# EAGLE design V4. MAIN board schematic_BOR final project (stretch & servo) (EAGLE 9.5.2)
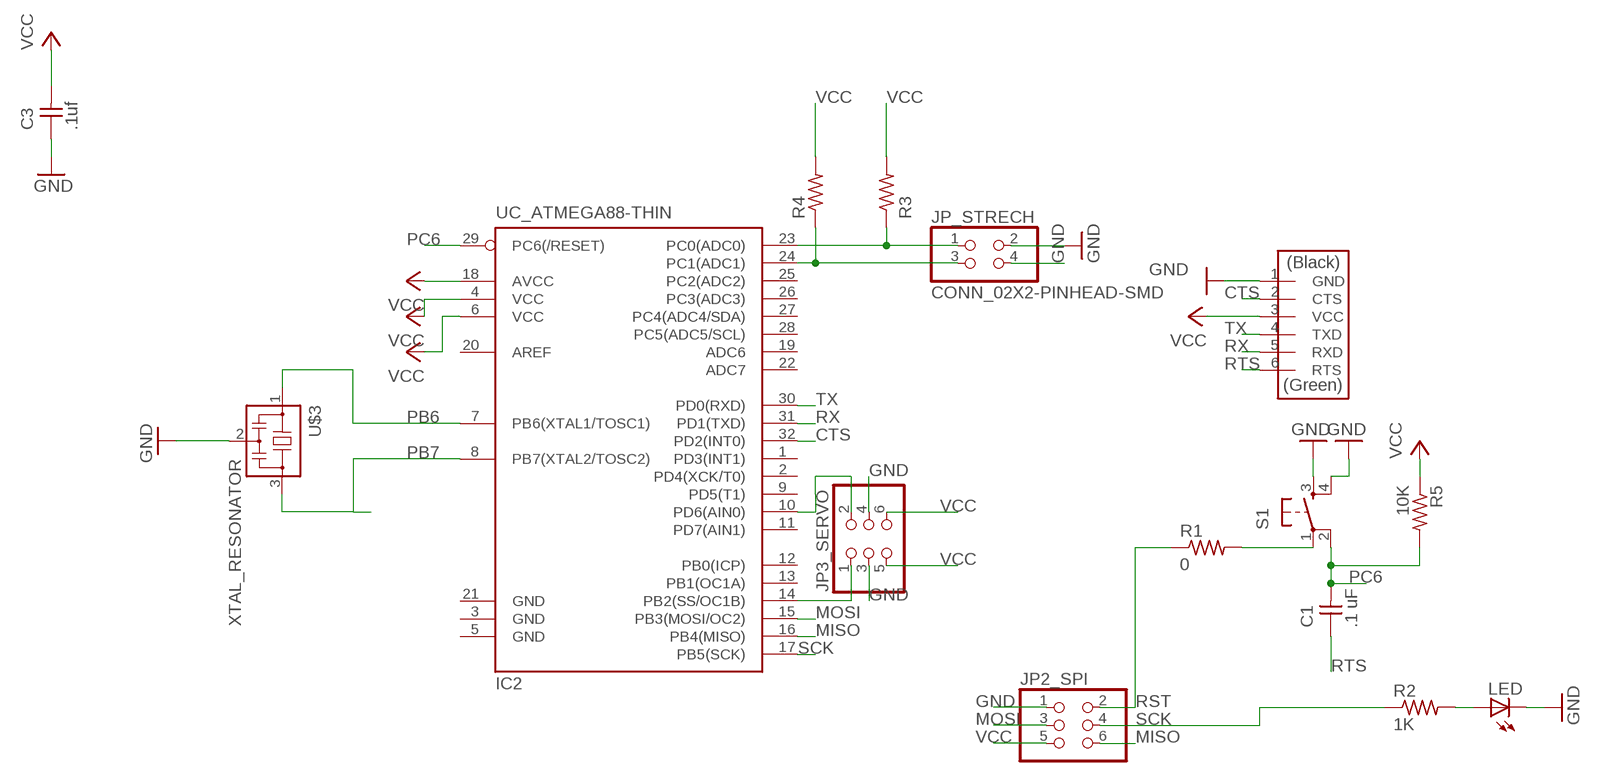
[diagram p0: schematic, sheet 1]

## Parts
C1  .1 uF  CAP_UNPOLARIZEDFAB  [C1206FAB]
C3  .1uf  UNPOLARIZED_CAPACITOR1206  [1206]
IC2  UC_ATMEGA88-THIN  [TQFP32-08THIN]
JP2_SPI  CONN_03X2-PINHEAD-SMD  [2X03SMD]
JP3_SERVO  CONN_03X2-PINHEAD-SMD  [2X03SMD]
JP_STRECH  CONN_02X2-PINHEAD-SMD  [2X02SMD]
LED  LED1206  [1206]
R1  0  R1206FAB  [R1206FAB]
R2  1K  RESISTOR1206  [1206]
R3  R1206FAB  [R1206FAB]
R4  R1206FAB  [R1206FAB]
R5  10K  RESISTOR1206  [1206]
S1  SW_SWITCH_TACTILE_6MM6MM_SWITCH  [6MM_SWITCH]
U$1  CONN_06_FTDI-SMD-HEADER  [1X06SMD]
U$3  XTAL_RESONATOR  [EFOBM]

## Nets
CTS: IC2.32(PD2(INT0)) U$1.2(CTS)
GND: C3.1 JP2_SPI.1 JP3_SERVO.3 JP3_SERVO.4 JP_STRECH.2 JP_STRECH.4 LED.2(C) S1.3(S) S1.4(S1) U$1.1(GND) U$3.2
MISO: IC2.16(PB4(MISO)) JP2_SPI.6
MOSI: IC2.15(PB3(MOSI/OC2)) JP2_SPI.3
N$1: R1.2 S1.1(P)
N$2: IC2.10(PD6(AIN0)) JP3_SERVO.2
N$3: IC2.23(PC0(ADC0)) JP_STRECH.1 R3.1
N$4: IC2.24(PC1(ADC1)) JP_STRECH.3 R4.1
N$18: IC2.14(PB2(SS/OC1B)) JP3_SERVO.1
N$23: LED.1(A) R2.2
PB6: IC2.7(PB6(XTAL1/TOSC1)) U$3.1
PB7: IC2.8(PB7(XTAL2/TOSC2)) U$3.3
PC6: C1.2 IC2.29(PC6(/RESET)) R5.2 S1.2(P1)
RST: JP2_SPI.2 R1.1
RTS: C1.1 U$1.6(RTS)
RX: IC2.31(PD1(TXD)) U$1.5(RXD)
SCK: IC2.17(PB5(SCK)) JP2_SPI.4 R2.1
TX: IC2.30(PD0(RXD)) U$1.4(TXD)
VCC: C3.2 IC2.4(VCC) IC2.6(VCC) IC2.18(AVCC) JP2_SPI.5 JP3_SERVO.5 JP3_SERVO.6 R3.2 R4.2 R5.1 U$1.3(VCC)
Unconnected: IC2.1(PD3(INT1)) IC2.2(PD4(XCK/T0)) IC2.9(PD5(T1)) IC2.11(PD7(AIN1)) IC2.12(PB0(ICP)) IC2.13(PB1(OC1A)) IC2.19(ADC6) IC2.20(AREF) IC2.22(ADC7) IC2.25(PC2(ADC2)) IC2.26(PC3(ADC3)) IC2.27(PC4(ADC4/SDA)) IC2.28(PC5(ADC5/SCL))

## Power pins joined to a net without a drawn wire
GND: IC2.3(GND) IC2.5(GND) IC2.21(GND)

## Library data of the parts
C1 = eagle_fab:CAP_UNPOLARIZED
C3 = ng:UNPOLARIZED_CAPACITOR: unpolarized_capacitor
IC2 = eagle_fab:UC_ATMEGA88-THIN
JP2_SPI JP3_SERVO = eagle_fab:CONN_03X2-PINHEAD-SMD: PIN HEADER
JP_STRECH = eagle_fab:CONN_02X2-PINHEAD-SMD
LED = ng:LED
R1 R3 R4 = eagle_fab:R: Resistor (US Symbol)
R2 R5 = ng:RESISTOR
S1 = eagle_fab:SW_SWITCH_TACTILE_6MM: OMRON SWITCH
U$1 = eagle_fab:CONN_06_FTDI-SMD-HEADER
U$3 = eagle_fab:XTAL_RESONATOR

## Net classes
0 default: clearance 0.356 mm

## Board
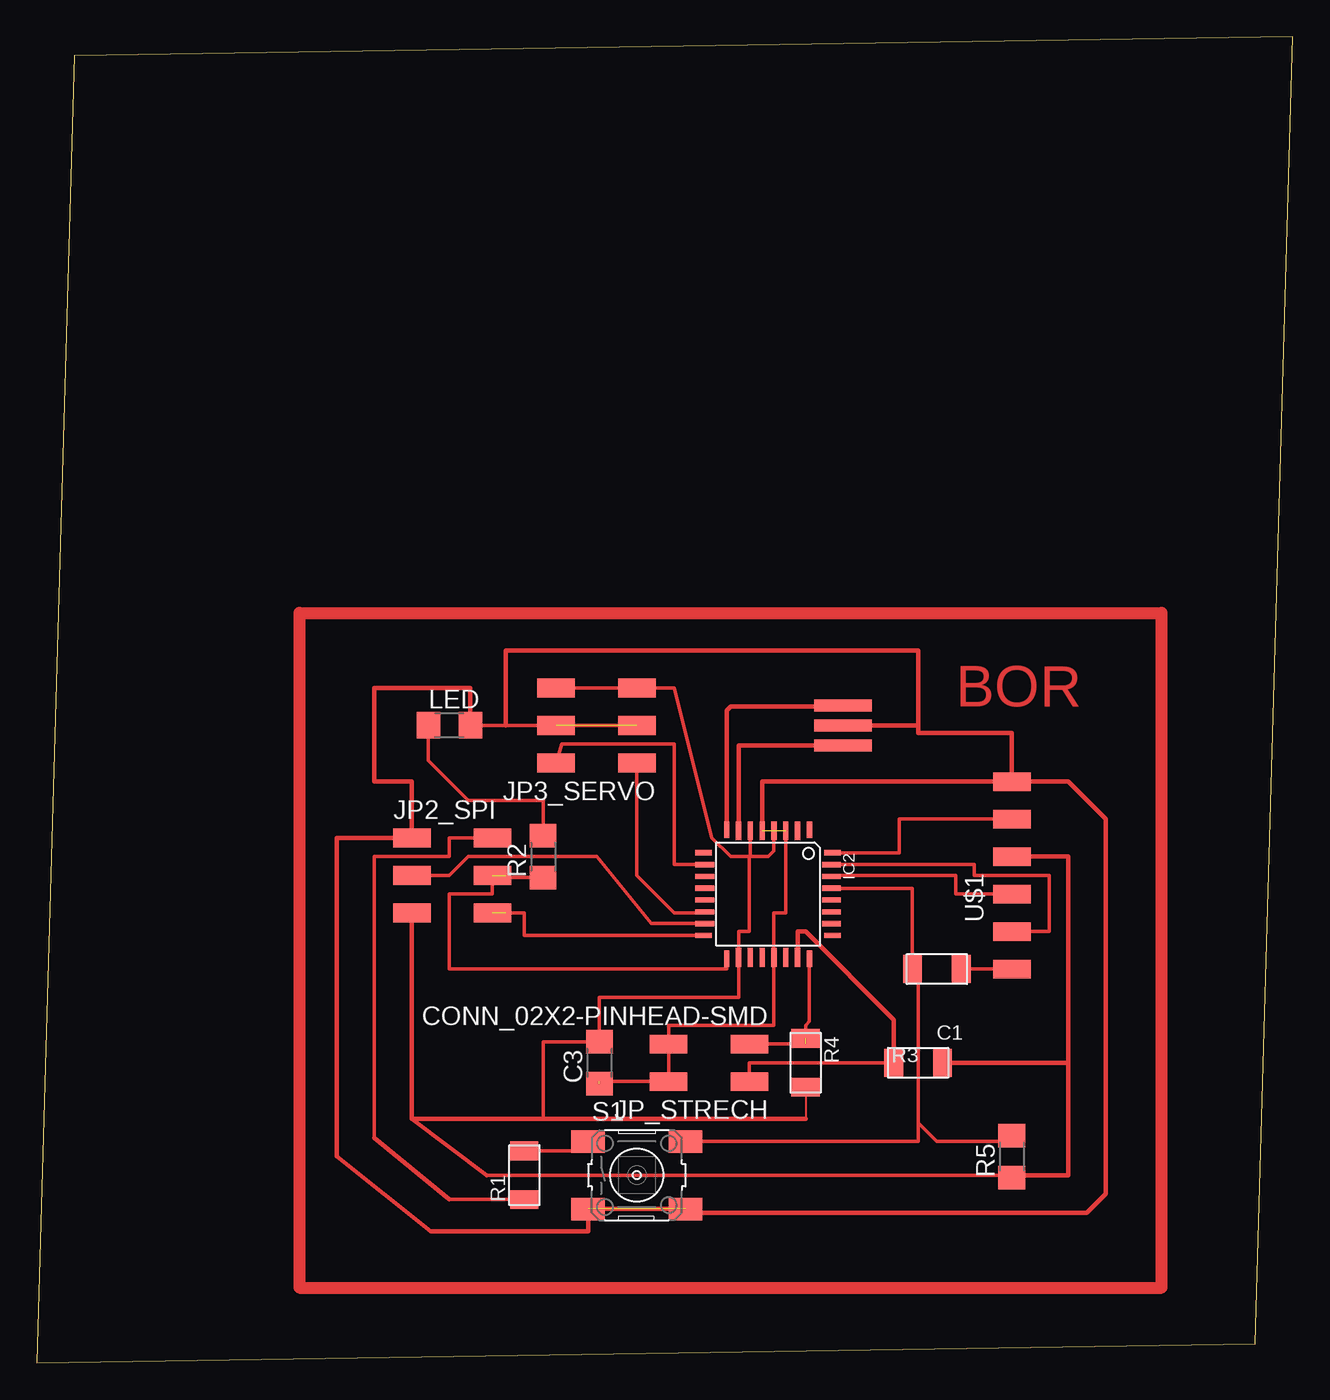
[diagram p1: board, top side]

Size 85.07 x 89.84 mm. Coordinates in mm from the lower left corner, seen from the top.
Outline: 0,0 82.53,1.27 85.07,89.84 2.54,88.57 0,0
Copper layers (1*16): Top 0.035mm / dielectric 1.5mm / Bottom 0.035mm
Design rules "default": minimum track width 6mil, minimum drill 0.35mm, track to track 6mil, track to pad 6mil, pad to pad 6mil, via to via 6mil, smd to smd 6mil, copper to edge 40mil, drill to drill 6mil, minimum pad ring 10mil, minimum via ring 8mil, stop-mask expansion 4mil, vias tented up to drill 0mil, thermal gap 10mil

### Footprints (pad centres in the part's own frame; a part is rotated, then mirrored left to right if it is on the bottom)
C1206FAB = smd 1.27 x 1.905: 1 -1.651,0; 2 1.651,0
1206 = smd 1.6 x 1.803: 1 -1.422,0; 2 1.422,0
TQFP32-08THIN = smd 1.118 x 0.356: 1 -4.369,2.8; 8 -4.369,-2.8; 17 4.369,-2.8; 24 4.369,2.8 | smd 1.27 x 0.356: 2 -4.293,2; 3 -4.293,1.2; 4 -4.293,0.4; 5 -4.293,-0.4; 6 -4.293,-1.2; 7 -4.293,-2; 18 4.293,-2; 19 4.293,-1.2; 20 4.293,-0.4; 21 4.293,0.4; 22 4.293,1.2; 23 4.293,2 | smd 0.356 x 1.118: 9 -2.8,-4.369; 16 2.8,-4.369; 25 2.8,4.369; 32 -2.8,4.369 | smd 0.356 x 1.27: 10 -2,-4.293; 14 1.2,-4.293; 15 2,-4.293; 26 2,4.293; 27 1.2,4.293; 31 -2,4.293 | smd 0.35 x 1.27: 11 -1.2,-4.293; 12 -0.4,-4.293; 13 0.4,-4.293; 28 0.4,4.293; 29 -0.4,4.293; 30 -1.2,4.293
2X03SMD = smd 2.54 x 1.27: 1 -2.54,2.54; 2 2.92,2.54; 3 -2.54,0; 4 2.92,0; 5 -2.54,-2.54; 6 2.92,-2.54
2X02SMD = smd 2.54 x 1.27: 1 -2.54,1.27; 2 2.92,1.27; 3 -2.54,-1.27; 4 2.92,-1.27
R1206FAB = smd 1.27 x 1.905: 1 -1.651,0; 2 1.651,0
6MM_SWITCH = smd 2.286 x 1.524: 1 -3.302,2.286; 2 3.302,2.286; 3 -3.302,-2.286; 4 3.302,-2.286
1X06SMD = smd 2.54 x 1.27: 1 0,6.35; 2 0,3.81; 3 0,1.27; 4 0,-1.27; 5 0,-3.81; 6 0,-6.35
EFOBM = smd 0.8 x 3.9: 1 -1.35,0; 2 0,0; 3 1.35,0

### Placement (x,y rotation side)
C1  60.96,26.67 180 top
C3  38.1,20.32 90 top
IC2  49.53,31.75 270 top
JP2_SPI  27.94,33.02 0 top
JP3_SERVO  38.1,43.18 180 top
JP_STRECH  45.72,20.32 180 top
LED  27.94,43.18 0 top
R1  33.02,12.7 90 top
R2  34.29,34.29 90 top
R3  59.69,20.32 0 top
R4  52.07,20.32 270 top
R5  66.04,13.97 90 top
S1  40.64,12.7 0 top
U$1  66.04,33.02 0 top
U$3  54.61,43.18 90 top

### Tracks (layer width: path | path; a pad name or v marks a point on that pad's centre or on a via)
CTS
  Top 0.254: U$1.2 58.42,36.83 58.42,34.55 IC2.32
GND  (4 unrouted)
  Top 0.152: 44.2,10.41 44.45,10.16
  Top 0.254: LED.2 31.75,43.18 JP3_SERVO.3 | 38.1,19.05 JP_STRECH.2 JP_STRECH.4 42.8,22.86 49.93,22.86 IC2.21 49.93,30.48 50.73,30.48 IC2.3
  Top 0.305: U$3.2 59.69,43.18 | IC2.5 49.13,39.37 U$1.1 66.04,42.67 59.69,42.67 59.69,43.18 | LED.2 29.36,45.72 22.86,45.72 22.86,39.37 25.4,39.37 JP2_SPI.1 20.32,35.56 20.32,13.97 26.67,8.89 37.34,8.89 S1.3 44.2,10.41 | 59.69,43.18 59.69,48.26 31.75,48.26 31.75,43.18 | 44.45,10.16 71.12,10.16 72.39,11.43 72.39,36.83 69.85,39.37 67.31,39.37
MISO  (1 unrouted)
  Top 0.254: IC2.16 33.02,28.95 33.02,30.48 31.75,30.48
MOSI
  Top 0.254: IC2.15 41.63,29.75 38.1,34.1 37.91,34.29 29.21,34.29 27.94,33.02 JP2_SPI.3
N$1
  Top 0.254: R1.2 37.34,14.35 S1.1
N$2
  Top 0.152: 41.91,41.91 41.91,41.89
  Top 0.254: JP3_SERVO.2 35.56,41.91 41.91,41.91 43.18,41.91 43.18,33.75 IC2.10
N$3  (1 unrouted)
  Top 0.152: 58.19,20.55 R3.1 | 58.15,20.49 57.98,20.32
  Top 0.254: JP_STRECH.1 48.26,20.32 57.98,20.32 | IC2.23 51.53,27.21
  Top 0.305: R3.1 58.04,23.24 52.07,29.21 51.53,29.21 IC2.23
N$4  (1 unrouted)
  Top 0.254: 52.07,21.59 JP_STRECH.3 | IC2.24 52.33,23.12 52.07,22.86 R4.1
N$5
  Top 0.813: 17.78,50.8 76.2,50.8 76.2,5.08 17.78,5.08 17.78,50.8
N$18
  Top 0.152: IC2.14 45.17,30.48
  Top 0.254: 45.17,30.48 43.18,30.48 40.64,33.02 JP3_SERVO.1
N$23
  Top 0.254: R2.2 34.29,38.1 29.21,38.1 26.52,40.79 LED.1
PB6
  Top 0.305: U$3.1 47.53,41.83 IC2.7
PB7
  Top 0.152: U$3.3 54.53,44.45
  Top 0.305: 54.53,44.45 46.99,44.45 46.73,44.19 IC2.8
PC6
  Top 0.152: 59.69,16.26 59.66,16.23 | 66.04,14.99 R5.2
  Top 0.254: 59.69,16.26 59.69,14.99 S1.2 | 59.69,16.26 60.96,14.99 66.04,14.99 | IC2.29 59.31,32.15 C1.2 59.69,26.67 59.69,16.26
RST
  Top 0.254: JP2_SPI.2 27.94,35.56 27.94,34.29 22.86,34.29 22.86,15.24 | 27.94,11.05 R1.1
  Top 0.305: 22.86,15.24 27.94,11.05
RTS
  Top 0.254: C1.1 U$1.6
RX
  Top 0.254: IC2.31 63.5,33.75 63.5,33.02 68.58,33.02 68.58,29.21 U$1.5
SCK  (1 unrouted)
  Top 0.152: 31.75,32.87 31.75,33.02
  Top 0.254: JP2_SPI.4 30.86,31.75 27.94,31.75 27.94,26.67 46.73,26.67 IC2.17 | R2.1 31.75,32.87
TX
  Top 0.152: IC2.30 53.82,33.02
  Top 0.254: 53.82,33.02 62.23,33.02 62.23,31.75 U$1.4
VCC
  Top 0.152: R4.2 52.07,16.51 | 66.19,12.7 R5.1 65.89,12.7
  Top 0.254: IC2.4 49.93,34.69 49.53,34.29 48.33,34.29 | 48.26,34.29 48.26,29.21 47.53,29.21 IC2.18 47.53,24.74 38.1,24.74 C3.2 34.29,21.74 34.29,16.51 | JP3_SERVO.6 JP3_SERVO.5 43.18,45.72 45.72,35.56 46.99,34.29 48.26,34.29 | 30.48,12.7 65.89,12.7 | IC2.6 48.33,34.29 | 48.33,34.29 48.26,34.29
  Top 0.305: U$1.3 69.85,34.29 69.85,20.32 | 69.85,20.32 69.85,12.7 66.19,12.7 | 25.4,16.51 JP2_SPI.5 | 25.4,16.51 34.29,16.51 52.07,16.51 | R3.2 69.85,20.32 | 25.4,16.51 30.48,12.7

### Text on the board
Top: BOR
